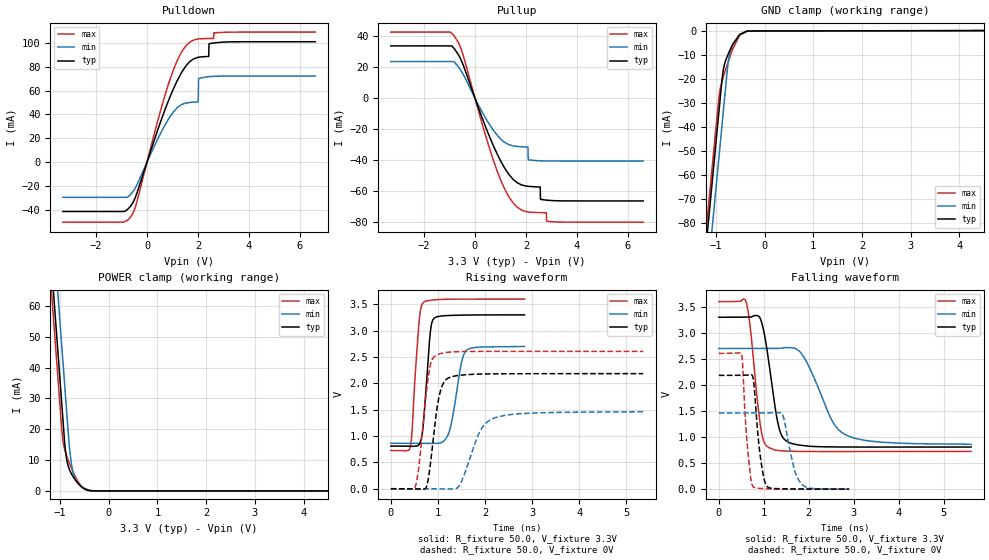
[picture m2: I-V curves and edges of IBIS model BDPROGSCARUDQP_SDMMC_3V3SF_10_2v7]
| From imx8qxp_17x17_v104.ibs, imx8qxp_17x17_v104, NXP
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[Model]   BDPROGSCARUDQP_SDMMC_3V3SF_10_2v7
Model_type I/O
Polarity   Non-Inverting
Enable   Active-Low
| CAP_THRESHOLD on pad IO is "CMOS" :
| Rising=10.0% of vdde3v3   Falling=90.0% of vdde3v3
| C_comp min and max val. don't necessarily correlate with the min and max pvt
| but are the smallest and greatest pad capacitance found.
| var   typ   min   max
C_comp   1.26795pF  1.18790pF  1.31090pF
Vinl = 675.0mV
Vinh = 2.25V
Vmeas = 1.65V   | Reference voltage for timing measurements
Cref  = 15.0pF   | Timing specification test load capacitance value
Rref  = 1.0MOhm   | Timing specification test load resistance value
Vref  = 3.3V   | Timing specification test load voltage
[Model Spec]
| TIME_THRESHOLD on pin ZI is "CORE" :
| Rising=50.0% of vdd   Falling=50.0% of vdd
Vinl 825.00000mV 675.00000mV 900.00000mV
Vinh 2.06250V 1.68750V 2.25000V
Vmeas 1.65000V 1.35000V 1.80000V
Vref 3.30000V 2.70000V 3.60000V
| variable   typ   min   max
[Temperature Range] 25.0 125.0 -40.0
| variable   typ   min   max
[Voltage Range] 3.3V 2.7V 3.6V
| variable   typ   min   max
[POWER Clamp Reference] 3.3V 2.7V 3.6V
| variable   typ   min   max
[GND Clamp Reference] 0V 0V 0V
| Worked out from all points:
|   slope of the pulldown table from 0 to 0.495 V, typ, clamps not added: 15.7 ohm
|   slope of the pullup table from 0 to 0.495 V, typ, clamps not added: 22.8 ohm
|   GND clamp passes 1 mA (typ) near -0.46 V on its own axis
|   POWER clamp passes 1 mA (typ) near -0.53 V on its own axis
|   rising waveform, R_fixture 50.0, V_fixture 3.3V: 20-80 % time 123ps typ, 204ps min, 122ps max; typ from 0.809 V to 3.3 V
|   falling waveform, R_fixture 50.0, V_fixture 3.3V: 20-80 % time 256ps typ, 562ps min, 203ps max; typ from 3.3 V to 0.809 V
|   rising waveform, R_fixture 50.0, V_fixture 0V: 20-80 % time 188ps typ, 376ps min, 183ps max; typ from 0 V to 2.18 V
|   falling waveform, R_fixture 50.0, V_fixture 0V: 20-80 % time 149ps typ, 220ps min, 122ps max; typ from 2.18 V to 0 V
[POWER Clamp]
-3.3V     524.6mA    543.4mA    516.1mA
-1.18V    74.13mA    92.92mA    65.73mA
-1.13V    63.5mA     82.3mA     55.11mA
-1.08V    52.88mA    71.67mA    44.49mA
-1.02V    40.13mA    58.93mA    31.74mA
-950mV    25.26mA    44.05mA    17.6mA
-900mV    14.93mA    33.43mA    13.17mA
-860mV    9.966mA    24.93mA    11.19mA
-800mV    6.661mA    13.12mA    8.673mA
-730mV    4.611mA    5.939mA    6.078mA
-460mV    377.7uA    598.1uA    338.7uA
6.6V      0A         0A         0A
[GND Clamp]
-3.3V     -535.9mA   -554.9mA   -529.5mA
-1.29V    -108.7mA   -127.8mA   -102.4mA
-1.13V    -74.74mA   -93.8mA    -68.39mA
-980mV    -42.86mA   -61.92mA   -36.51mA
-940mV    -34.36mA   -53.42mA   -28.08mA
-870mV    -19.62mA   -38.55mA   -20.84mA
-840mV    -15.5mA    -32.17mA   -18.78mA
-750mV    -9.826mA   -13.7mA    -13.06mA
-690mV    -7.205mA   -7.371mA   -9.546mA
-510mV    -1.433mA   -1.699mA   -1.633mA
-360mV    -54.77uA   -166.3uA   -42.24uA
6.6V      207.7uA    166.8uA    268.6uA
| variable   typ   min   max
[Pullup Reference] 3.3V 2.7V 3.6V
| variable   typ   min   max
[Pulldown Reference] 0V 0V 0V
[Pullup]
-3.3V     33.71mA    23.63mA    42.63mA
-820mV    32.13mA    23.52mA    40.3mA
-490mV    22.58mA    16.21mA    29.14mA
880mV     -36.28mA   -24.03mA   -47.35mA
1.65V     -54.46mA   -31.12mA   -70.18mA
2.08V     -56.83mA   -31.54mA   -73.39mA
2.1V      -56.87mA   -39.77mA   -73.43mA
2.56V     -57.29mA   -40.39mA   -73.82mA
2.58V     -65.28mA   -40.4mA    -73.83mA
2.8V      -65.75mA   -40.48mA   -73.9mA
2.82V     -65.78mA   -40.48mA   -79.42mA
6.6V      -66.28mA   -40.54mA   -79.99mA
[Pulldown]
-3.3V     -41.49mA   -29.63mA   -50.48mA
-670mV    -37.68mA   -27.73mA   -46.92mA
-430mV    -28.08mA   -20.54mA   -35.73mA
880mV     53.64mA    37.35mA    68.04mA
1.67V     84.2mA     50.02mA    100.6mA
2.01V     87.93mA    50.5mA     103.3mA
2.02V     87.97mA    68.44mA    103.4mA
2.12V     88.28mA    70.63mA    103.5mA
2.42V     88.69mA    71.69mA    103.7mA
2.43V     99.17mA    71.71mA    103.7mA
2.63V     100mA      72.01mA    108.5mA
6.6V      101mA      72.22mA    109.1mA
[Ramp]
dV/dt_r 1.3099V/188.25171ps 876.03737mV/376.35625ps 1.5632V/183.30229ps
dV/dt_f 1.49389V/256.0841ps 1.10217V/561.72092ps 1.72452V/202.50135ps
R_load = 50.0
| Removed startup time: 0s 0s 0s  .
| Removed end time: 2.82ns.
[Rising Waveform]
R_fixture   = 50.0
V_fixture   = 3.3V
V_fixture_min = 2.7V
V_fixture_max = 3.6V
0s        808.7mV    861.9mV    724mV
410ps     808mV      861.9mV    780mV
450ps     804.2mV    861.9mV    1.075V
590ps     827.9mV    861.9mV    3.062V
680ps     1.133V     861.9mV    3.522V
830ps     2.89V      858.5mV    3.575V
910ps     3.225V     859.8mV    3.583V
1.23ns    3.287V     1.053V     3.595V
1.6ns     3.295V     2.618V     3.597V
2.84ns    3.299V     2.699V     3.598V
| Removed startup time: 0s 0s 0s  .
| Removed end time: 5.59ns.
[Falling Waveform]
R_fixture   = 50.0
V_fixture   = 3.3V
V_fixture_min = 2.7V
V_fixture_max = 3.6V
0s        3.299V     2.699V     3.598V
610ps     3.302V     2.699V     3.591V
930ps     3.26V      2.699V     1.202V
1.11ns    2.457V     2.7V       800.7mV
1.34ns    1.176V     2.701V     740.1mV
1.58ns    890.3mV    2.715V     728.4mV
1.89ns    835.1mV    2.537V     723.4mV
2.52ns    810.8mV    1.312V     722.4mV
2.81ns    808.9mV    1.049V     722.7mV
5.61ns    808.7mV    861.9mV    724mV
| Removed startup time: 0s 0s 0s  .
| Removed end time: 5.34ns.
[Rising Waveform]
R_fixture   = 50.0
V_fixture   = 0V
V_fixture_min = 0V
V_fixture_max = 0V
0s        118.5uV    97.08uV    137.3uV
520ps     -4.522mV   160.1uV    39.01mV
770ps     73.97mV    -576.7uV   1.938V
850ps     536.9mV    -2.117mV   2.39V
970ps     1.462V     -2.156mV   2.534V
1.2ns     2.09V      -4.462mV   2.588V
1.46ns    2.152V     66.05mV    2.601V
1.89ns    2.175V     1.084V     2.605V
2.2ns     2.179V     1.343V     2.606V
5.36ns    2.183V     1.46V      2.605V
| Removed startup time: 0s 0s 0s  .
| Removed end time: 2.88ns.
[Falling Waveform]
R_fixture   = 50.0
V_fixture   = 0V
V_fixture_min = 0V
V_fixture_max = 0V
0s        2.183V     1.46V      2.605V
510ps     2.185V     1.46V      2.589V
630ps     2.188V     1.461V     894mV
770ps     2.105V     1.462V     44.11mV
920ps     653.7mV    1.462V     12.7mV
1.07ns    54.57mV    1.464V     6.523mV
1.42ns    5.985mV    1.423V     2.094mV
1.68ns    3.311mV    376.5mV    683.3uV
1.86ns    2.368mV    87.05mV    346.6uV
2.9ns     118.5uV    96.68uV    137.4uV
